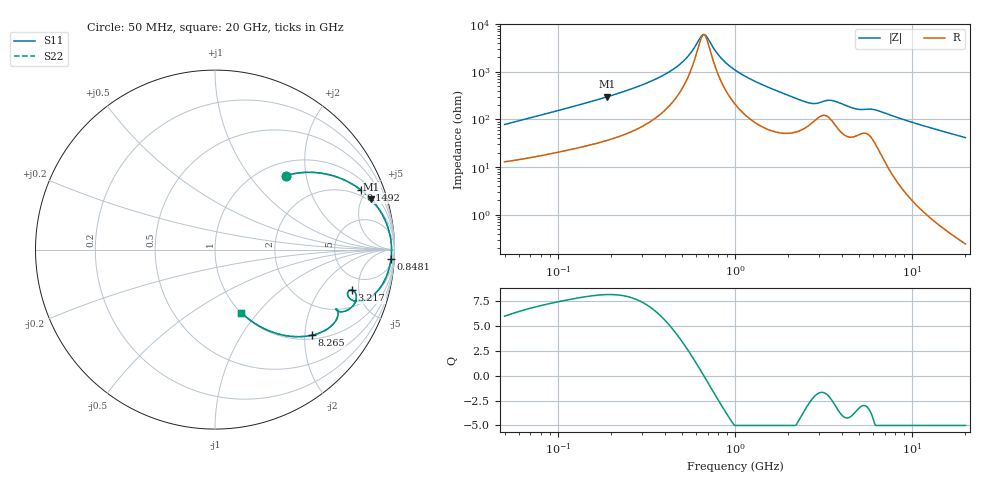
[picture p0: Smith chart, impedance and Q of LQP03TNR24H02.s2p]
!Murata Part Number: LQP03TNR24H02
!These Parameters are Measured in Series Mode Connection
!  o--[Z]--o
!Port1  Port2
!  o-------o
!Freq. Start=50[MHz] Stop=20[GHz], 401[Steps]
# Hz S RI R 50
!Freq.(Hz) S11(Real) S11(Imag) S21(Real) S21(Imag) S12(Real) S12(Imag) S22(Real) S22(Imag)
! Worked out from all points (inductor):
!   401 points, 50 MHz to 20 GHz, reference 50 ohm
!   read as one part in series: L = 241 nH near 51.52 MHz
!   highest Q = 8.15 at 189.6 MHz (marker M1), where L = 247 nH
!   self-resonance near 657.4 MHz
!   S11 on the Smith chart (normalised r, x): 50 MHz: 1.26, +1.54; 149.2 MHz: 1.57, +4.54; 848.1 MHz: 12, -35; 3.217 GHz: 3.42, -4.23; 8.265 GHz: 1.10, -2.18; 20 GHz: 1.00, -0.83
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5e7  0.3948 0.4123  0.6052 -0.4123  0.6052 -0.4123  0.3948 0.4123
8.074856e7  0.5927 0.4256  0.4073 -0.4256  0.4073 -0.4256  0.5927 0.4256
1.364002e8  0.7851 0.3522  0.2149 -0.3522  0.2149 -0.3522  0.7851 0.3522
1.492265e8  0.8114 0.3335  0.1886 -0.3335  0.1886 -0.3335  0.8114 0.3335
1.896393e8  0.8708 0.2796  0.1292 -0.2796  0.1292 -0.2796  0.8708 0.2796
3.721004e8  0.9635 0.1233  0.0365 -0.1233  0.0365 -0.1233  0.9635 0.1233
5.096456e8  0.9794 0.0558  0.0206 -0.0558  0.0206 -0.0558  0.9794 0.0558
6.574395e8  0.9837 0.00285  0.0163 -0.00285  0.0163 -0.00285  0.9837 0.00285
6.87656e8  0.9837 -0.00649  0.0163 0.00649  0.0163 0.00649  0.9837 -0.00649
8.480927e8  0.9809 -0.0507  0.0191 0.0507  0.0191 0.0507  0.9809 -0.0507
1e9  0.9748 -0.0868  0.0252 0.0868  0.0252 0.0868  0.9748 -0.0868
1.639343e9  0.9236 -0.2076  0.0764 0.2076  0.0764 0.2076  0.9236 -0.2076
2.279204e9  0.8272 -0.2842  0.1728 0.2842  0.1728 0.2842  0.8272 -0.2842
2.728004e9  0.7482 -0.2699  0.2518 0.2699  0.2518 0.2699  0.7482 -0.2699
3.216634e9  0.764 -0.226  0.236 0.226  0.236 0.226  0.764 -0.226
3.792786e9  0.7824 -0.2902  0.2176 0.2902  0.2176 0.2902  0.7824 -0.2902
4.608136e9  0.7065 -0.3461  0.2935 0.3461  0.2935 0.3461  0.7065 -0.3461
5.598765e9  0.6808 -0.3346  0.3192 0.3346  0.3192 0.3346  0.6808 -0.3346
7.442007e9  0.603 -0.4556  0.397 0.4556  0.397 0.4556  0.603 -0.4556
8.264682e9  0.5418 -0.4769  0.4582 0.4769  0.4582 0.4769  0.5418 -0.4769
1.314879e10  0.2937 -0.4496  0.7063 0.4496  0.7063 0.4496  0.2937 -0.4496
2e10  0.1475 -0.3517  0.8525 0.3517  0.8525 0.3517  0.1475 -0.3517
